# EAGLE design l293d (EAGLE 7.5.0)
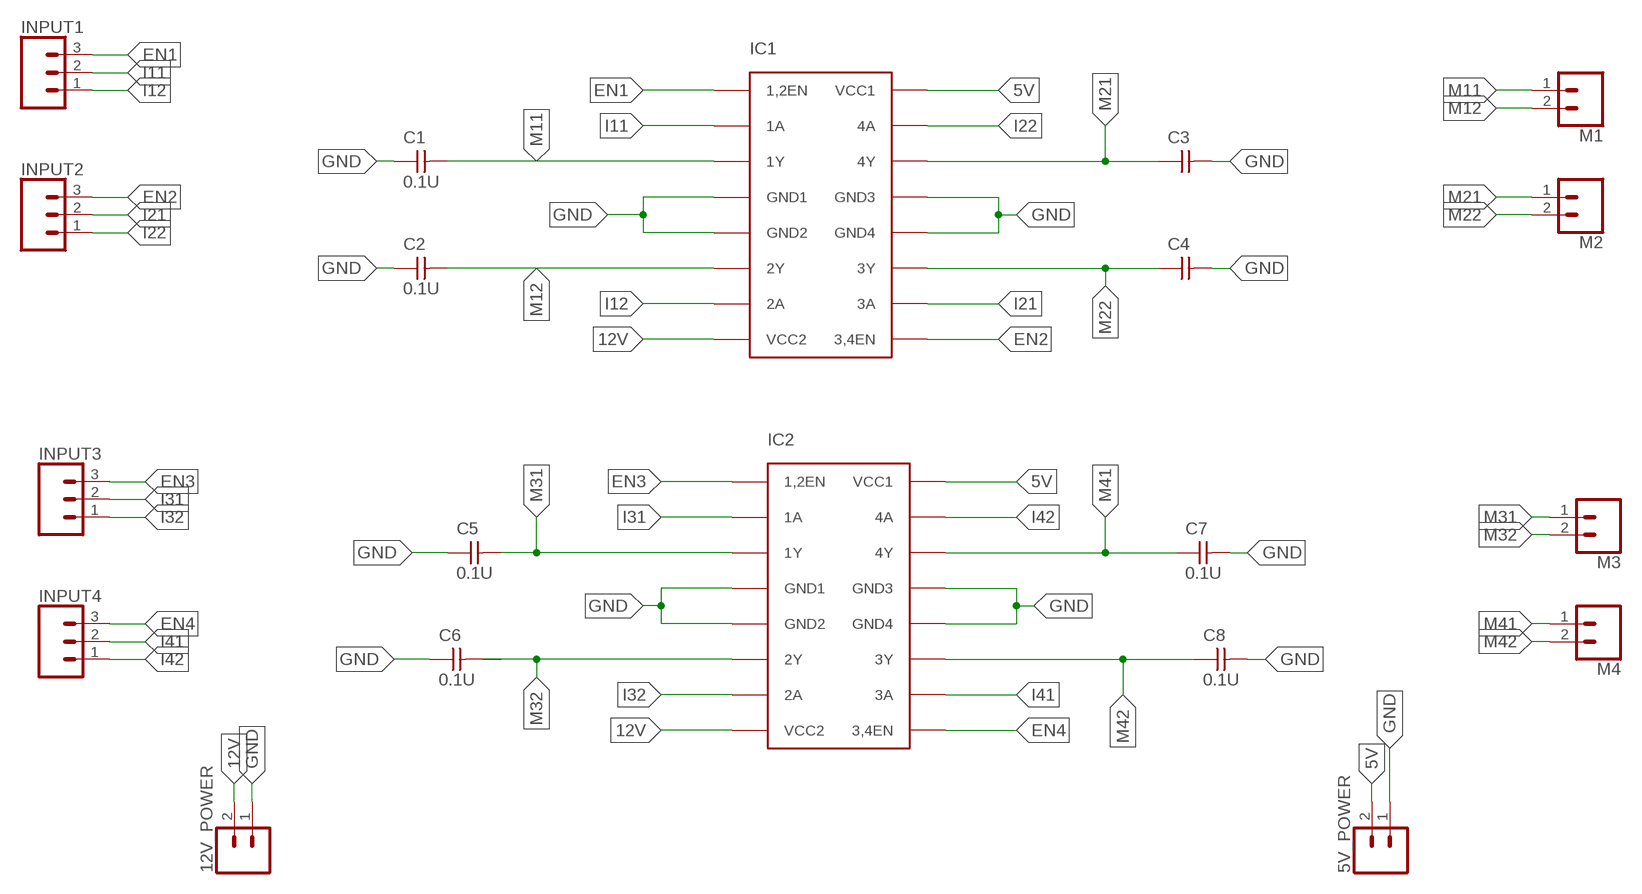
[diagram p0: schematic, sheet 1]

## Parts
5V_POWER  CONN_02LOCK  [1X02_LOCK]
12V_POWER  CONN_02LOCK  [1X02_LOCK]
C1  0.1U  CAP-UNPOLARIZEDFAB  [C1206FAB]
C2  0.1U  CAP-UNPOLARIZEDFAB  [C1206FAB]
C3  CAP-UNPOLARIZEDFAB  [C1206FAB]
C4  CAP-UNPOLARIZEDFAB  [C1206FAB]
C5  0.1U  CAP-UNPOLARIZEDFAB  [C1206FAB]
C6  0.1U  CAP-UNPOLARIZEDFAB  [C1206FAB]
C7  0.1U  CAP-UNPOLARIZEDFAB  [C1206FAB]
C8  0.1U  CAP-UNPOLARIZEDFAB  [C1206FAB]
IC1  L293D  [DIL16]
IC2  L293D  [DIL16]
INPUT1  CONN_03LOCK  [1X03_LOCK]
INPUT2  CONN_03LOCK  [1X03_LOCK]
INPUT3  CONN_03LOCK  [1X03_LOCK]
INPUT4  CONN_03LOCK  [1X03_LOCK]
M1  CONN_02LOCK  [1X02_LOCK]
M2  CONN_02LOCK  [1X02_LOCK]
M3  CONN_02LOCK  [1X02_LOCK]
M4  CONN_02LOCK  [1X02_LOCK]

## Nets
5V: 5V_POWER.2 IC1.16(VCC1) IC2.16(VCC1)
12V: 12V_POWER.2 IC1.8(VCC2) IC2.8(VCC2)
EN1: IC1.1(1,2EN) INPUT1.3
EN2: IC1.9(3,4EN) INPUT2.3
EN3: IC2.1(1,2EN) INPUT3.3
EN4: IC2.9(3,4EN) INPUT4.3
GND: 5V_POWER.1 12V_POWER.1 C1.1 C2.1 C3.2 C4.2 C5.1 C6.1 C7.2 C8.2 IC1.4(GND1) IC1.5(GND2) IC1.12(GND4) IC1.13(GND3) IC2.4(GND1) IC2.5(GND2) IC2.12(GND4) IC2.13(GND3)
I11: IC1.2(1A) INPUT1.2
I12: IC1.7(2A) INPUT1.1
I21: IC1.10(3A) INPUT2.2
I22: IC1.15(4A) INPUT2.1
I31: IC2.2(1A) INPUT3.2
I32: IC2.7(2A) INPUT3.1
I41: IC2.10(3A) INPUT4.2
I42: IC2.15(4A) INPUT4.1
M11: C1.2 IC1.3(1Y) M1.1
M12: C2.2 IC1.6(2Y) M1.2
M21: C3.1 IC1.14(4Y) M2.1
M22: C4.1 IC1.11(3Y) M2.2
M31: C5.2 IC2.3(1Y) M3.1
M32: C6.2 IC2.6(2Y) M3.2
M41: C7.1 IC2.14(4Y) M4.1
M42: C8.1 IC2.11(3Y) M4.2

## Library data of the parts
5V_POWER 12V_POWER M1-M4 = SparkFun-Connectors:CONN_02: Multi connection point. Often used as Generic Header-pin footprint for 0.1 inch spaced/style header connections
C1-C8 = fab:CAP-UNPOLARIZED
IC1 IC2 = h-bridge:L293D
INPUT1-INPUT4 = SparkFun-Connectors:CONN_03: Multi connection point. Often used as Generic Header-pin footprint for 0.1 inch spaced/style header connections On any of the 0.1 inch spaced packages, you can populate with these: Break Away Headers - Straight (PRT-00116) Break Away Male Headers - Right Angle (PRT-00553) Female Headers (PRT-00115)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

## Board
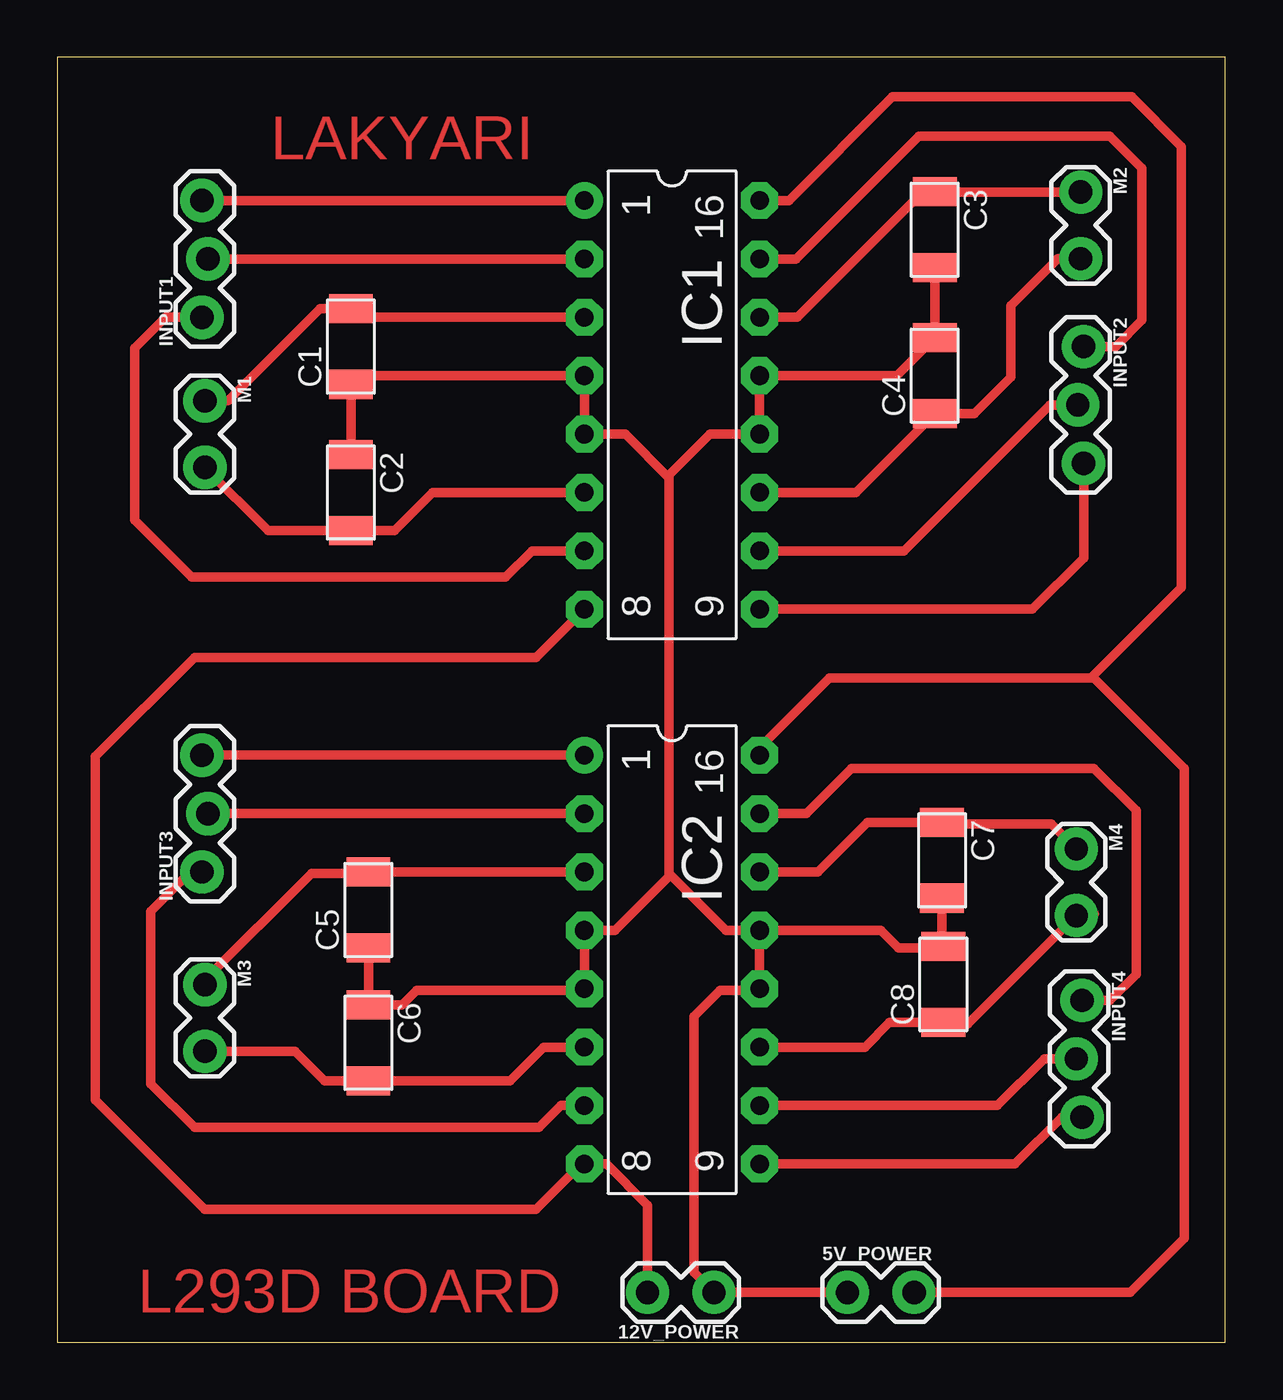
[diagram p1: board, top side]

Size 50.8 x 55.88 mm. Coordinates in mm from the lower left corner, seen from the top.
Outline: 0,0 50.8,0 50.8,55.88 0,55.88 0,0
Copper layers (1*16): Top 0.035mm / dielectric 1.5mm / Bottom 0.035mm
Design rules "default": minimum track width 10mil, minimum drill 24mil, track to track 8mil, track to pad 8mil, pad to pad 8mil, via to via 8mil, smd to smd 8mil, copper to edge 40mil, drill to drill 8mil, minimum pad ring 10mil, minimum via ring 8mil, stop-mask expansion 4mil, vias tented up to drill 0mil, thermal gap 10mil

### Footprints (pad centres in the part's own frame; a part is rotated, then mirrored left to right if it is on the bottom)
1X02_LOCK = drill 1.016 pad 1.88: 1 -0.178,0; 2 2.718,0
C1206FAB = smd 1.27 x 1.905: 1 -1.651,0; 2 1.651,0
DIL16 = drill 0.813 pad 1.6: 1 -8.89,-3.81 | drill 0.813 pad 1.6 octagon: 2 -6.35,-3.81; 3 -3.81,-3.81; 4 -1.27,-3.81; 5 1.27,-3.81; 6 3.81,-3.81; 7 6.35,-3.81; 8 8.89,-3.81; 9 8.89,3.81; 10 6.35,3.81; 11 3.81,3.81; 12 1.27,3.81; 13 -1.27,3.81; 14 -3.81,3.81; 15 -6.35,3.81; 16 -8.89,3.81
1X03_LOCK = drill 1.016 pad 1.88: 1 0,0.127; 2 2.54,-0.127; 3 5.08,0.127

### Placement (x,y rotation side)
5V_POWER  34.54,2.16 0 top
12V_POWER  28.38,2.16 180 top
C1  12.76,43.31 90 top
C2  12.76,36.96 270 top
C3  38.16,48.39 270 top
C4  38.16,42.04 90 top
C5  13.53,18.8 90 top
C6  13.53,13.02 270 top
C7  38.48,20.95 270 top
C8  38.54,15.56 90 top
IC1  26.73,40.77 270 top
IC2  26.73,16.64 270 top
INPUT1  6.41,44.58 90 top
INPUT2  44.51,43.31 270 top
INPUT3  6.41,20.45 90 top
INPUT4  44.45,14.86 270 top
M1  6.41,40.77 270 top
M2  44.51,49.85 270 top
M3  6.41,15.37 270 top
M4  44.32,21.27 270 top

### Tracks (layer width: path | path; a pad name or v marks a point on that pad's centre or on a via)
5V
  Top 0.406: IC1.16 31.81,49.66 36.32,54.17 46.74,54.17 48.9,52.01 48.9,32.83 44.96,28.89 | IC2.16 30.54,25.84 33.59,28.89 44.96,28.89 | 5V_POWER.2 46.67,2.16 49.02,4.51 49.02,24.96 45.09,28.89 44.96,28.89
12V
  Top 0.406: 12V_POWER.2 25.67,5.96 23.88,7.75 IC2.8 22.8,7.75 20.83,5.78 6.41,5.78 1.65,10.54 1.65,25.46 5.97,29.78 20.83,29.78 IC1.8
EN1
  Top 0.406: INPUT1.3 IC1.1
EN2
  Top 0.406: INPUT2.3 44.64,34.1 42.42,31.88 IC1.9
EN3
  Top 0.406: INPUT3.3 IC2.1
EN4
  Top 0.406: IC2.9 41.66,7.75 43.69,9.78 INPUT4.3
GND
  Top 0.406: C2.1 C1.1 13.14,42.04 IC1.4 IC1.5 24.7,39.5 26.61,37.59 | C3.2 C4.2 36.51,42.04 IC1.13 IC1.12 28.38,39.5 26.61,37.72 26.61,37.59 | 26.61,37.59 26.61,20.38 | 26.61,20.38 26.61,20.26 24.26,17.91 IC2.4 IC2.5 22.86,15.3 15.62,15.3 14.99,14.67 C6.1 | 13.59,14.61 C6.1 | C5.1 C6.1 | IC2.13 IC2.12 30.48,15.3 28.83,15.3 27.69,14.16 27.69,3.04 12V_POWER.1 5V_POWER.1 | C7.2 38.48,17.27 C8.2 38.48,17.14 36.58,17.14 35.81,17.91 IC2.13 | IC2.13 29.08,17.91 26.61,20.38
I11
  Top 0.406: IC1.2 INPUT1.2
I12
  Top 0.406: INPUT1.1 4.7,44.58 3.37,43.24 3.37,35.75 5.84,33.27 19.49,33.27 20.64,34.42 IC1.7
I21
  Top 0.406: IC1.10 36.83,34.42 43.18,40.77 INPUT2.2
I22
  Top 0.406: INPUT2.1 46.04,43.31 47.18,44.45 47.18,51.05 45.78,52.45 37.47,52.45 32.13,47.12 IC1.15
I31
  Top 0.406: INPUT3.2 IC2.2
I32
  Top 0.406: INPUT3.1 5.78,20.45 4.06,18.73 4.06,11.24 5.97,9.34 20.95,9.34 21.91,10.29 IC2.7
I41
  Top 0.406: IC2.10 40.89,10.29 42.93,12.32 INPUT4.2
I42
  Top 0.406: IC2.15 32.58,22.99 34.54,24.96 45.09,24.96 46.93,23.11 46.93,16 45.78,14.86 INPUT4.1
M11
  Top 0.406: IC1.3 13.14,44.58 C1.2 11.43,44.96 7.43,40.96 6.43,40.96 M1.1
M12
  Top 0.406: M1.2 9.16,35.31 C2.2 14.67,35.31 16.32,36.96 IC1.6
M21
  Top 0.406: M2.1 38.18,50.02 C3.1 37.66,50.04 32.19,44.58 IC1.14
M22
  Top 0.406: M2.2 43.51,47.13 41.47,45.09 41.47,41.97 39.88,40.39 C4.1 34.73,36.96 IC1.11
M31
  Top 0.406: IC2.3 C5.2 13.46,20.38 11.05,20.38 6.41,15.75 M3.1
M32
  Top 0.406: M3.2 10.34,12.65 11.62,11.37 C6.2 19.68,11.37 21.14,12.83 IC2.6
M41
  Top 0.406: IC2.14 33.08,20.45 35.24,22.61 C7.1 38.54,22.54 43.23,22.54 M4.1
M42
  Top 0.406: 45.1,18.62 M4.2 39.61,13.84 38.61,13.84 C8.1 36.2,13.91 35.12,12.83 IC2.11

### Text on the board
Top: LAKYARI | L293D BOARD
